| IBIS file stm32wba63_a65_ufbga121_smps_usb.ibs
[IBIS ver] 4.2
[File name] stm32wba63_a65_ufbga121_smps_usb.ibs
[File Rev] 2.0
[Date] 17-02-2025
[Source] Data Created at STMicroelectronics
[Notes]  File originated from ELDO simulations.
[Disclaimer]  This information is for modeling purpose only and is
   not guaranted. The information is subject to change without
   notice.
[Copyright] Copyright 2025 STMicroelectronics Inc.
|   Component stm32wba63_a65_ufbga121_smps_usb
[Component] stm32wba63_a65_ufbga121_smps_usb
[Manufacturer] STMicroelectronics
[Package]
| variable   typ   min   max
R_pkg  0  NA  NA
L_pkg  0  NA  NA
C_pkg  0  NA  NA
[Pin]   signal_name   model_name
A1  PD10  io8_ft_100m
A10  VSSRF  nc
A11 RF  nc
A2  PD11  io8_ft_100m
A3  PD13  io8_ft_100m_i2c
A4  PC2  io8_ft_100m
A5  VDD11  nc
A6  VDD  power
A7  VDDRFPA  nc
A8  OSC_IN  nc
A9  VDDRF  nc
B1  VDDSMPS  nc
B10  VSSRF  nc
B11  NRST  ioreset_v33
B2  PB13  io8_ft_100m_i2c
B3  PB14  io8_ft_100m_i2c
B4  PA9  io8_ft_100m
B5  PC5  io8_ft_100m
B6  VSS  gnd
B7  VDDHPA  nc
B8  OSC_OUT  nc
B9  VDDANA  nc
C1  VLXSMPS  nc
C10  VSS  gnd
C11  VDD  power
C2  VSSSMPS  nc
C3  VDD  power
C4  PD12  io8_ft_100m_i2c
C5  PC4  io8_ft_100m
C6  PC3  io8_ft_100m
C7  VSSRF  nc
C8  VSSRF  nc
C9  PH3-BOOT0  io8_ft_100m_v33
D1  PB11  io8_ft_100m_i2c
D10  PB2  io8_ft_100m_i2c_v33
D11  PC6  io8_ft_100m
D2  PA8  io8_ft_100m
D3  VSS  gnd
D4  PB12  io8_ft_100m
D5  PA7  io8_ft_100m_i2c_v33
D6  PA10  io8_ft_100m
D7  PA14  io8_ft_100m_v33
D8  PB15  io8_ft_100m
D9  PA13  io8_ft_100m
E1  VREFP  nc
E10  PC10  io8_ft_100m
E11  PC9  io8_ft_100m
E2  VSSA  nc
E3  PA6  io8_ft_100m_i2c
E4  PC0  io8_ft_100m_i2c
E5  PA5  io8_ft_100m
E6  PE0  io8_ft_100m_hslv
E7  PC11  io8_ft_100m
E8  PC7  io8_ft_100m
E9  PC8  io8_ft_100m
F1  VDDA  nc
F10  PB0  io8_ft_100m
F11  PB1  io8_ft_100m_i2c
F2  PC1  io8_ft_100m_i2c
F3  PA3  io8_ft_100m
F4  PD9  io8_ft_100m
F5  PD4  io8_ft_100m
F6  PE3  io8_ft_100m_hslv
F7  PE1  io8_ft_100m_hslv
F8  PC12  io8_ft_100m
F9  PA11  io8_ft_100m
G1  PA4  io8_ft_100m_v33
G10  VSS  gnd
G11  VDD  power
G2  PB10  io8_ft_100m_i2c
G3  PA2  io8_ft_100m_v33
G4  PD8  io8_ft_100m
G5  PG10  io8_ft_100m_hslv
G6  VSS  gnd
G7  PG5  io8_ft_100m_hslv
G8  PE2  io8_ft_100m_hslv
G9  PA12  io8_ft_100m
H1  PA1  io8_ft_100m
H10  PD14  io8_ft_100m_hslv
H11  PB3  io8_ft_100m_i2c
H2  PA0  io8_ft_100m
H3  VSS  gnd
H4  PD3  io8_ft_100m
H5  PD0  io8_ft_100m
H6  VDDIO2  power
H7  PG6  io8_ft_100m_hslv
H8  PE6  io8_ft_100m
H9  PA15  io8_ft_100m_i2c
J1  PB9  io8_ft_100m
J10  PB4  io8_ft_100m
J11  VSS  gnd
J2  VDD  power
J3  VSS  gnd
J4  PD1  io8_ft_100m
J5  PD15  io8_ft_100m
J6  PG13  io8_ft_100m_hslv
J7  PG9  io8_ft_100m_hslv
J8  PG3  io8_ft_100m_hslv
J9  PE5  io8_ft_100m
K1  VDDUSB  power
K10  PE4  io8_ft_100m
K11  VDD  power
K2  PD6  io8_ft_100m
K3  PB8  io8_ft_100m
K4  PC14-OSC32_IN  io_ft_tamp
K5  PG15  io8_ft_100m_hslv
K6  PG11  io8_ft_100m_hslv
K7  PG8  io8_ft_100m_hslv
K8  PG2  io8_ft_100m_hslv
K9  PB7  io8_ft_100m
L1  PD7  io8_ft_100m
L10  PB6  io8_ft_100m
L11  PB5  io8_ft_100m
L2  PD5  io8_ft_100m
L3  PD2  io8_ft_100m
L4  PC15-OSC32_OUT  io_ft_tamp
L5  PG14  io8_ft_100m_hslv
L6  PG12  io8_ft_100m_hslv
L7  PG7  io8_ft_100m_hslv
L8  PG4  io8_ft_100m_hslv
L9  PC13  io8_ft_100m_v33
[Package Model]   4b0-ufbga-6x6-121-241118
[Pin Mapping]   pulldown_ref   pullup_ref   | Comment
A1  gndio  vddio
A10  nc  nc
A11  nc  nc
A2  gndio  vddio
A3  gndio  vddio
A4  gndio  vddio
A5  nc  nc
A6  nc  vddio
A7  nc  nc
A8  nc  nc
A9  nc  nc
B1  nc  nc
B10  nc  nc
B11  gndio  vddio
B2  gndio  vddio
B3  gndio  vddio
B4  gndio  vddio
B5  gndio  vddio
B6  gndio  nc
B7  nc  nc
B8  nc  nc
B9  nc  nc
C1  nc  nc
C10  gndio  nc
C11  nc  vddio
C2  nc  nc
C3  nc  vddio
C4  gndio  vddio
C5  gndio  vddio
C6  gndio  vddio
C7  nc  nc
C8  nc  nc
C9  gndio  vddio
D1  gndio  vddio
D10  gndio  vddio
D11  gndio  vddio
D2  gndio  vddio
D3  gndio  nc
D4  gndio  vddio
D5  gndio  vddio
D6  gndio  vddio
D7  gndio  vddio
D8  gndio  vddio
D9  gndio  vddio
E1  nc  nc
E10  gndio  vddio
E11  gndio  vddio
E2  nc  nc
E3  gndio  vddio
E4  gndio  vddio
E5  gndio  vddio
E6  gndio  vddio
E7  gndio  vddio
E8  gndio  vddio
E9  gndio  vddio
F1  nc  nc
F10  gndio  vddio
F11  gndio  vddio
F2  gndio  vddio
F3  gndio  vddio
F4  gndio  vddio  | Depending on IO usage
| F4  gndio  vddusb  | Depending on IO usage
F5  gndio  vddio
F6  gndio  vddio
F7  gndio  vddio
F8  gndio  vddio
F9  gndio  vddio
G1  gndio  vddio
G10  gndio  nc
G11  nc  vddio
G2  gndio  vddio
G3  gndio  vddio
G4  gndio  vddio  | Depending on IO usage
| G4  gndio  vddusb  | Depending on IO usage
G5  gndio  vddio2
G6  gndio  nc
G7  gndio  vddio2
G8  gndio  vddio
G9  gndio  vddio
H1  gndio  vddio
H10  gndio  vddio
H11  gndio  vddio
H2  gndio  vddio
H3  gndio  nc
H4  gndio  vddio
H5  gndio  vddio
H6  nc  vddio2
H7  gndio  vddio2
H8  gndio  vddio
H9  gndio  vddio
J1  gndio  vddio
J10  gndio  vddio
J11  gndio  nc
J2  nc  vddio
J3  gndio  nc
J4  gndio  vddio
J5  gndio  vddio
J6  gndio  vddio2
J7  gndio  vddio2
J8  gndio  vddio2
J9  gndio  vddio
K1  nc  vddusb
K10  gndio  vddio
K11  nc  vddio
K2  gndio  vddio
K3  gndio  vddio
K4  gndio  vddio
K5  gndio  vddio2
K6  gndio  vddio2
K7  gndio  vddio2
K8  gndio  vddio2
K9  gndio  vddio
L1  gndio  vddio
L10  gndio  vddio
L11  gndio  vddio
L2  gndio  vddio
L3  gndio  vddio
L4  gndio  vddio
L5  gndio  vddio2
L6  gndio  vddio2
L7  gndio  vddio2
L8  gndio  vddio2
L9  gndio  vddio
|[Diff Pin]  inv_pin  vdiff  tdelay_typ  tdelay_min  tdelay_max
|K2  L1  NA  NA  NA  NA
[Model Selector] io8_ft_100m
io8_ft_100m_ls_1v2  "GPIO 100MHz - 5V tolerant - low speed - 1.2V range"
io8_ft_100m_ls_1v8  "GPIO 100MHz - 5V tolerant - low speed - 1.8V range"
io8_ft_100m_ls_3v3  "GPIO 100MHz - 5V tolerant - low speed - 3.3V range"
io8_ft_100m_ms_1v2  "GPIO 100MHz - 5V tolerant - med speed - 1.2V range"
io8_ft_100m_ms_1v8  "GPIO 100MHz - 5V tolerant - med speed - 1.8V range"
io8_ft_100m_ms_3v3  "GPIO 100MHz - 5V tolerant - med speed - 3.3V range"
io8_ft_100m_fs_1v2  "GPIO 100MHz - 5V tolerant - fast speed - 1.2V range"
io8_ft_100m_fs_1v8  "GPIO 100MHz - 5V tolerant - fast speed - 1.8V range"
io8_ft_100m_fs_3v3  "GPIO 100MHz - 5V tolerant - fast speed - 3.3V range"
io8_ft_100m_hs_1v2  "GPIO 100MHz - 5V tolerant - high speed - 1.2V range"
io8_ft_100m_hs_1v8  "GPIO 100MHz - 5V tolerant - high speed - 1.8V range"
io8_ft_100m_hs_3v3  "GPIO 100MHz - 5V tolerant - high speed - 3.3V range"
[Model Selector] io8_ft_100m_hslv
io8_ft_100m_ls_1v2  "GPIO 100MHz - 5V tolerant - low speed - 1.2V range"
io8_ft_100m_ls_1v8  "GPIO 100MHz - 5V tolerant - low speed - 1.8V range"
io8_ft_100m_ls_3v3  "GPIO 100MHz - 5V tolerant - low speed - 3.3V range"
io8_ft_100m_ms_1v2  "GPIO 100MHz - 5V tolerant - med speed - 1.2V range"
io8_ft_100m_ms_1v8  "GPIO 100MHz - 5V tolerant - med speed - 1.8V range"
io8_ft_100m_ms_3v3  "GPIO 100MHz - 5V tolerant - med speed - 3.3V range"
io8_ft_100m_fs_1v2  "GPIO 100MHz - 5V tolerant - fast speed - 1.2V range"
io8_ft_100m_fs_1v8  "GPIO 100MHz - 5V tolerant - fast speed - 1.8V range"
io8_ft_100m_fs_3v3  "GPIO 100MHz - 5V tolerant - fast speed - 3.3V range"
io8_ft_100m_hs_1v2  "GPIO 100MHz - 5V tolerant - high speed - 1.2V range"
io8_ft_100m_hs_1v8  "GPIO 100MHz - 5V tolerant - high speed - 1.8V range"
io8_ft_100m_hs_3v3  "GPIO 100MHz - 5V tolerant - high speed - 3.3V range"
io8_ft_100m_hslv_ls_1v2  "GPIO 100MHz lv opt - 5V tolerant - low speed - 1.2V range"
io8_ft_100m_hslv_ls_1v8  "GPIO 100MHz lv opt - 5V tolerant - low speed - 1.8V range"
io8_ft_100m_hslv_ls_2v5  "GPIO 100MHz lv opt - 5V tolerant - low speed - 2.5V range"
io8_ft_100m_hslv_ms_1v2  "GPIO 100MHz lv opt - 5V tolerant - med speed - 1.2V range"
io8_ft_100m_hslv_ms_1v8  "GPIO 100MHz lv opt - 5V tolerant - med speed - 1.8V range"
io8_ft_100m_hslv_ms_2v5  "GPIO 100MHz lv opt - 5V tolerant - med speed - 2.5V range"
io8_ft_100m_hslv_fs_1v2  "GPIO 100MHz lv opt - 5V tolerant - fast speed - 1.2V range"
io8_ft_100m_hslv_fs_1v8  "GPIO 100MHz lv opt - 5V tolerant - fast speed - 1.8V range"
io8_ft_100m_hslv_fs_2v5  "GPIO 100MHz lv opt - 5V tolerant - fast speed - 2.5V range"
io8_ft_100m_hslv_hs_1v2  "GPIO 100MHz lv opt - 5V tolerant - high speed - 1.2V range"
io8_ft_100m_hslv_hs_1v8  "GPIO 100MHz lv opt - 5V tolerant - high speed - 1.8V range"
io8_ft_100m_hslv_hs_2v5  "GPIO 100MHz lv opt - 5V tolerant - high speed - 2.5V range"
[Model Selector] io8_ft_100m_i2c
io8_ft_100m_ls_1v2  "GPIO 100MHz - 5V tolerant - low speed - 1.2V range"
io8_ft_100m_ls_1v8  "GPIO 100MHz - 5V tolerant - low speed - 1.8V range"
io8_ft_100m_ls_3v3  "GPIO 100MHz - 5V tolerant - low speed - 3.3V range"
io8_ft_100m_ms_1v2  "GPIO 100MHz - 5V tolerant - med speed - 1.2V range"
io8_ft_100m_ms_1v8  "GPIO 100MHz - 5V tolerant - med speed - 1.8V range"
io8_ft_100m_ms_3v3  "GPIO 100MHz - 5V tolerant - med speed - 3.3V range"
io8_ft_100m_fs_1v2  "GPIO 100MHz - 5V tolerant - fast speed - 1.2V range"
io8_ft_100m_fs_1v8  "GPIO 100MHz - 5V tolerant - fast speed - 1.8V range"
io8_ft_100m_fs_3v3  "GPIO 100MHz - 5V tolerant - fast speed - 3.3V range"
io8_ft_100m_hs_1v2  "GPIO 100MHz - 5V tolerant - high speed - 1.2V range"
io8_ft_100m_hs_1v8  "GPIO 100MHz - 5V tolerant - high speed - 1.8V range"
io8_ft_100m_hs_3v3  "GPIO 100MHz - 5V tolerant - high speed - 3.3V range"
io8_ft_100m_i2c_ls_1v2  "GPIO 100MHz with I2C open-drain - 5V tolerant - low speed - 1.2V range"
io8_ft_100m_i2c_ls_1v8  "GPIO 100MHz with I2C open-drain - 5V tolerant - low speed - 1.8V range"
io8_ft_100m_i2c_ls_3v3  "GPIO 100MHz with I2C open-drain - 5V tolerant - low speed - 3.3V range"
io8_ft_100m_i2c_ms_1v2  "GPIO 100MHz with I2C open-drain - 5V tolerant - med speed - 1.2V range"
io8_ft_100m_i2c_ms_1v8  "GPIO 100MHz with I2C open-drain - 5V tolerant - med speed - 1.8V range"
io8_ft_100m_i2c_ms_3v3  "GPIO 100MHz with I2C open-drain - 5V tolerant - med speed - 3.3V range"
io8_ft_100m_i2c_fs_1v2  "GPIO 100MHz with I2C open-drain - 5V tolerant - fast speed - 1.2V range"
io8_ft_100m_i2c_fs_1v8  "GPIO 100MHz with I2C open-drain - 5V tolerant - fast speed - 1.8V range"
io8_ft_100m_i2c_fs_3v3  "GPIO 100MHz with I2C open-drain - 5V tolerant - fast speed - 3.3V range"
io8_ft_100m_i2c_hs_1v2  "GPIO 100MHz with I2C open-drain - 5V tolerant - high speed - 1.2V range"
io8_ft_100m_i2c_hs_1v8  "GPIO 100MHz with I2C open-drain - 5V tolerant - high speed - 1.8V range"
io8_ft_100m_i2c_hs_3v3  "GPIO 100MHz with I2C open-drain - 5V tolerant - high speed - 3.3V range"
io8_ft_100m_i2c_fmp_3v3  "GPIO 100MHz with I2C fm+ open-drain - 5V tolerant - low speed - 3.3V range"
io8_ft_100m_i2c_fmp_1v8  "GPIO 100MHz with I2C fm+ open-drain - 5V tolerant - low speed - 1.8V range"
io8_ft_100m_i2c_fmp_1v2  "GPIO 100MHz with I2C fm+ open-drain - 5V tolerant - low speed - 1.2V range"
[Model Selector] io8_ft_100m_i2c_v33
io8_ft_100m_v33_ls_1v2  "GPIO_V33 100MHz - 5V tolerant - low speed - 1.2V range"
io8_ft_100m_v33_ls_1v8  "GPIO_V33 100MHz - 5V tolerant - low speed - 1.8V range"
io8_ft_100m_v33_ls_3v3  "GPIO_V33 100MHz - 5V tolerant - low speed - 3.3V range"
io8_ft_100m_v33_ms_1v2  "GPIO_V33 100MHz - 5V tolerant - med speed - 1.2V range"
io8_ft_100m_v33_ms_1v8  "GPIO_V33 100MHz - 5V tolerant - med speed - 1.8V range"
io8_ft_100m_v33_ms_3v3  "GPIO_V33 100MHz - 5V tolerant - med speed - 3.3V range"
io8_ft_100m_v33_fs_1v2  "GPIO_V33 100MHz - 5V tolerant - fast speed - 1.2V range"
io8_ft_100m_v33_fs_1v8  "GPIO_V33 100MHz - 5V tolerant - fast speed - 1.8V range"
io8_ft_100m_v33_fs_3v3  "GPIO_V33 100MHz - 5V tolerant - fast speed - 3.3V range"
io8_ft_100m_v33_hs_1v2  "GPIO_V33 100MHz - 5V tolerant - high speed - 1.2V range"
io8_ft_100m_v33_hs_1v8  "GPIO_V33 100MHz - 5V tolerant - high speed - 1.8V range"
io8_ft_100m_v33_hs_3v3  "GPIO_V33 100MHz - 5V tolerant - high speed - 3.3V range"
io8_ft_100m_i2c_v33_ls_1v2  "GPIO_V33 100MHz with I2C open-drain - 5V tolerant - low speed - 1.2V range"
io8_ft_100m_i2c_v33_ls_1v8  "GPIO_V33 100MHz with I2C open-drain - 5V tolerant - low speed - 1.8V range"
io8_ft_100m_i2c_v33_ls_3v3  "GPIO_V33 100MHz with I2C open-drain - 5V tolerant - low speed - 3.3V range"
io8_ft_100m_i2c_v33_ms_1v2  "GPIO_V33 100MHz with I2C open-drain - 5V tolerant - med speed - 1.2V range"
io8_ft_100m_i2c_v33_ms_1v8  "GPIO_V33 100MHz with I2C open-drain - 5V tolerant - med speed - 1.8V range"
io8_ft_100m_i2c_v33_ms_3v3  "GPIO_V33 100MHz with I2C open-drain - 5V tolerant - med speed - 3.3V range"
io8_ft_100m_i2c_v33_fs_1v2  "GPIO_V33 100MHz with I2C open-drain - 5V tolerant - fast speed - 1.2V range"
io8_ft_100m_i2c_v33_fs_1v8  "GPIO_V33 100MHz with I2C open-drain - 5V tolerant - fast speed - 1.8V range"
io8_ft_100m_i2c_v33_fs_3v3  "GPIO_V33 100MHz with I2C open-drain - 5V tolerant - fast speed - 3.3V range"
io8_ft_100m_i2c_v33_hs_1v2  "GPIO_V33 100MHz with I2C open-drain - 5V tolerant - high speed - 1.2V range"
io8_ft_100m_i2c_v33_hs_1v8  "GPIO_V33 100MHz with I2C open-drain - 5V tolerant - high speed - 1.8V range"
io8_ft_100m_i2c_v33_hs_3v3  "GPIO_V33 100MHz with I2C open-drain - 5V tolerant - high speed - 3.3V range"
io8_ft_100m_i2c_fmp_v33_1v2  "GPIO_V33 100MHz with I2C fm+ open-drain - 5V tolerant - low speed - 1.2V range"
io8_ft_100m_i2c_fmp_v33_1v8  "GPIO_V33 100MHz with I2C fm+ open-drain - 5V tolerant - low speed - 1.8V range"
io8_ft_100m_i2c_fmp_v33_3v3  "GPIO_V33 100MHz with I2C fm+ open-drain - 5V tolerant - low speed - 3.3V range"
[Model Selector] io8_ft_100m_v33
io8_ft_100m_v33_ls_1v2  "GPIO_V33 100MHz - 5V tolerant - low speed - 1.2V range"
io8_ft_100m_v33_ls_1v8  "GPIO_V33 100MHz - 5V tolerant - low speed - 1.8V range"
io8_ft_100m_v33_ls_3v3  "GPIO_V33 100MHz - 5V tolerant - low speed - 3.3V range"
io8_ft_100m_v33_ms_1v2  "GPIO_V33 100MHz - 5V tolerant - med speed - 1.2V range"
io8_ft_100m_v33_ms_1v8  "GPIO_V33 100MHz - 5V tolerant - med speed - 1.8V range"
io8_ft_100m_v33_ms_3v3  "GPIO_V33 100MHz - 5V tolerant - med speed - 3.3V range"
io8_ft_100m_v33_fs_1v2  "GPIO_V33 100MHz - 5V tolerant - fast speed - 1.2V range"
io8_ft_100m_v33_fs_1v8  "GPIO_V33 100MHz - 5V tolerant - fast speed - 1.8V range"
io8_ft_100m_v33_fs_3v3  "GPIO_V33 100MHz - 5V tolerant - fast speed - 3.3V range"
io8_ft_100m_v33_hs_1v2  "GPIO_V33 100MHz - 5V tolerant - high speed - 1.2V range"
io8_ft_100m_v33_hs_1v8  "GPIO_V33 100MHz - 5V tolerant - high speed - 1.8V range"
io8_ft_100m_v33_hs_3v3  "GPIO_V33 100MHz - 5V tolerant - high speed - 3.3V range"
[Model Selector] io_ft_tamp
io_ft_tamp_ls_1v2 "io8_ft tamp low speed @ 1.2V"
io_ft_tamp_ls_1v8 "io8_ft tamp low speed @ 1.8V"
io_ft_tamp_ls_3v3 "io8_ft tamp low speed @ 3.3V"
io_ft_tamp_ms_1v2 "io8_ft tamp med speed @ 1.2V"
io_ft_tamp_ms_1v8 "io8_ft tamp med speed @ 1.8V"
io_ft_tamp_ms_3v3 "io8_ft tamp med speed @ 3.3V"
io_ft_tamp_fs_1v2 "io8_ft tamp fast speed @ 1.2V"
io_ft_tamp_fs_1v8 "io8_ft tamp fast speed @ 1.8V"
io_ft_tamp_fs_3v3 "io8_ft tamp fast speed @ 3.3V"
io_ft_tamp_hs_1v2 "io8_ft tamp high speed @ 1.2V"
io_ft_tamp_hs_1v8 "io8_ft tamp high speed @ 1.8V"
io_ft_tamp_hs_3v3 "io8_ft tamp high speed @ 3.3V"
[Model Selector] ioreset_v33
ioreset_v33_1v2 "Reset PAD. 5V tolerant. 1.2V range"
ioreset_v33_1v8 "Reset PAD. 5V tolerant. 1.8V range"
ioreset_v33_3v3 "Reset PAD. 5V tolerant. 3.3V range"
[Define Package Model]  4b0-ufbga-6x6-121-241118
[Manufacturer]  unknown
[OEM]  unknown
[Description]  unknown
[Number Of Pins]  106
[Pin Numbers]
| Pin Name Terminal   Net Name   Starting Node   Ending Node
A11 | RF
B11 | NRST
A8 | OSC_IN
B8 | OSC_OUT
H2 | PA0
H1 | PA1
G3 | PA2
F3 | PA3
G1 | PA4
E5 | PA5
E3 | PA6
D5 | PA7
D2 | PA8
B4 | PA9
D6 | PA10
F9 | PA11
G9 | PA12
D9 | PA13
D7 | PA14
H9 | PA15
F10 | PB0
F11 | PB1
D10 | PB2
H11 | PB3
J10 | PB4
L11 | PB5
L10 | PB6
K9 | PB7
K3 | PB8
J1 | PB9
G2 | PB10
D1 | PB11
D4 | PB12
B2 | PB13
B3 | PB14
D8 | PB15
E4 | PC0
F2 | PC1
A4 | PC2
C6 | PC3
C5 | PC4
B5 | PC5
D11 | PC6
E8 | PC7
E9 | PC8
E11 | PC9
E10 | PC10
E7 | PC11
F8 | PC12
L9 | PC13
K4 | PC14-OSC32_IN
L4 | PC15-OSC32_OUT
H5 | PD0
J4 | PD1
L3 | PD2
H4 | PD3
F5 | PD4
L2 | PD5
K2 | PD6
L1 | PD7
G4 | PD8
F4 | PD9
A1 | PD10
A2 | PD11
C4 | PD12
A3 | PD13
H10 | PD14
J5 | PD15
E6 | PE0
F7 | PE1
G8 | PE2
F6 | PE3
K10 | PE4
J9 | PE5
H8 | PE6
K8 | PG2
J8 | PG3
L8 | PG4
G7 | PG5
H7 | PG6
L7 | PG7
K7 | PG8
J7 | PG9
G5 | PG10
K6 | PG11
L6 | PG12
J6 | PG13
L5 | PG14
K5 | PG15
C9 | PH3-BOOT0
A5 | VDD11
A6 | VDD
F1 | VDDA
B9 | VDDANA
B7 | VDDHPA
H6 | VDDIO2
A9 | VDDRF
A7 | VDDRFPA
B1 | VDDSMPS
K1 | VDDUSB
C1 | VLXSMPS
E1 | VREFP
B6 | VSS
E2 | VSSA
A10 | VSSRF
C2 | VSSSMPS
|[Merged Pins]  B6
|C10  |  VSS
|D3  |  VSS
|G10  |  VSS
|G6  |  VSS
|H3  |  VSS
|J11  |  VSS
|J3  |  VSS
|[Merged Pins]  A6
|C11  |  VDD
|C3  |  VDD
|G11  |  VDD
|J2  |  VDD
|K11  |  VDD
|[Merged Pins]  A10
|B10  |  VSSRF
|C7  |  VSSRF
|C8  |  VSSRF
[Model Data]
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[End Model Data]
[End Package Model]
|End [Component]
| Models and submodels in the file (81): io8_ft_100m_fs_1v2 (I/O), io8_ft_100m_fs_1v8 (I/O), io8_ft_100m_fs_3v3 (I/O), io8_ft_100m_hs_1v2 (I/O), io8_ft_100m_hs_1v8 (I/O), io8_ft_100m_hs_3v3 (I/O), io8_ft_100m_hslv_fs_1v2 (I/O), io8_ft_100m_hslv_fs_1v8 (I/O), io8_ft_100m_hslv_fs_2v5 (I/O), io8_ft_100m_hslv_hs_1v2 (I/O), io8_ft_100m_hslv_hs_1v8 (I/O), io8_ft_100m_hslv_hs_2v5 (I/O), io8_ft_100m_hslv_ls_1v2 (I/O), io8_ft_100m_hslv_ls_1v8 (I/O), io8_ft_100m_hslv_ls_2v5 (I/O), io8_ft_100m_hslv_ms_1v2 (I/O), io8_ft_100m_hslv_ms_1v8 (I/O), io8_ft_100m_hslv_ms_2v5 (I/O), io8_ft_100m_i2c_fmp_1v2 (I/O_open_drain), io8_ft_100m_i2c_fmp_1v8 (I/O_open_drain), io8_ft_100m_i2c_fmp_3v3 (I/O_open_drain), io8_ft_100m_i2c_fmp_v33_1v2 (I/O_open_drain), io8_ft_100m_i2c_fmp_v33_1v8 (I/O_open_drain), io8_ft_100m_i2c_fmp_v33_3v3 (I/O_open_drain), io8_ft_100m_i2c_fs_1v2 (I/O_open_drain), io8_ft_100m_i2c_fs_1v8 (I/O_open_drain), io8_ft_100m_i2c_fs_3v3 (I/O_open_drain), io8_ft_100m_i2c_hs_1v2 (I/O_open_drain), io8_ft_100m_i2c_hs_1v8 (I/O_open_drain), io8_ft_100m_i2c_hs_3v3 (I/O_open_drain), io8_ft_100m_i2c_ls_1v2 (I/O_open_drain), io8_ft_100m_i2c_ls_1v8 (I/O_open_drain), io8_ft_100m_i2c_ls_3v3 (I/O_open_drain), io8_ft_100m_i2c_ms_1v2 (I/O_open_drain), io8_ft_100m_i2c_ms_1v8 (I/O_open_drain), io8_ft_100m_i2c_ms_3v3 (I/O_open_drain), io8_ft_100m_i2c_v33_fs_1v2 (I/O_open_drain), io8_ft_100m_i2c_v33_fs_1v8 (I/O_open_drain), io8_ft_100m_i2c_v33_fs_3v3 (I/O_open_drain), io8_ft_100m_i2c_v33_hs_1v2 (I/O_open_drain), io8_ft_100m_i2c_v33_hs_1v8 (I/O_open_drain), io8_ft_100m_i2c_v33_hs_3v3 (I/O_open_drain), io8_ft_100m_i2c_v33_ls_1v2 (I/O_open_drain), io8_ft_100m_i2c_v33_ls_1v8 (I/O_open_drain), io8_ft_100m_i2c_v33_ls_3v3 (I/O_open_drain), io8_ft_100m_i2c_v33_ms_1v2 (I/O_open_drain), io8_ft_100m_i2c_v33_ms_1v8 (I/O_open_drain), io8_ft_100m_i2c_v33_ms_3v3 (I/O_open_drain), io8_ft_100m_ls_1v2 (I/O), io8_ft_100m_ls_1v8 (I/O), io8_ft_100m_ls_3v3 (I/O), io8_ft_100m_ms_1v2 (I/O), io8_ft_100m_ms_1v8 (I/O), io8_ft_100m_ms_3v3 (I/O), io8_ft_100m_v33_fs_1v2 (I/O), io8_ft_100m_v33_fs_1v8 (I/O), io8_ft_100m_v33_fs_3v3 (I/O), io8_ft_100m_v33_hs_1v2 (I/O), io8_ft_100m_v33_hs_1v8 (I/O), io8_ft_100m_v33_hs_3v3 (I/O), io8_ft_100m_v33_ls_1v2 (I/O), io8_ft_100m_v33_ls_1v8 (I/O), io8_ft_100m_v33_ls_3v3 (I/O), io8_ft_100m_v33_ms_1v2 (I/O), io8_ft_100m_v33_ms_1v8 (I/O), io8_ft_100m_v33_ms_3v3 (I/O), io_ft_tamp_fs_1v2 (I/O), io_ft_tamp_fs_1v8 (I/O), io_ft_tamp_fs_3v3 (I/O), io_ft_tamp_hs_1v2 (I/O), io_ft_tamp_hs_1v8 (I/O), io_ft_tamp_hs_3v3 (I/O), io_ft_tamp_ls_1v2 (I/O), io_ft_tamp_ls_1v8 (I/O), io_ft_tamp_ls_3v3 (I/O), io_ft_tamp_ms_1v2 (I/O), io_ft_tamp_ms_1v8 (I/O), io_ft_tamp_ms_3v3 (I/O), ioreset_v33_1v2 (I/O_open_drain), ioreset_v33_1v8 (I/O_open_drain)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
